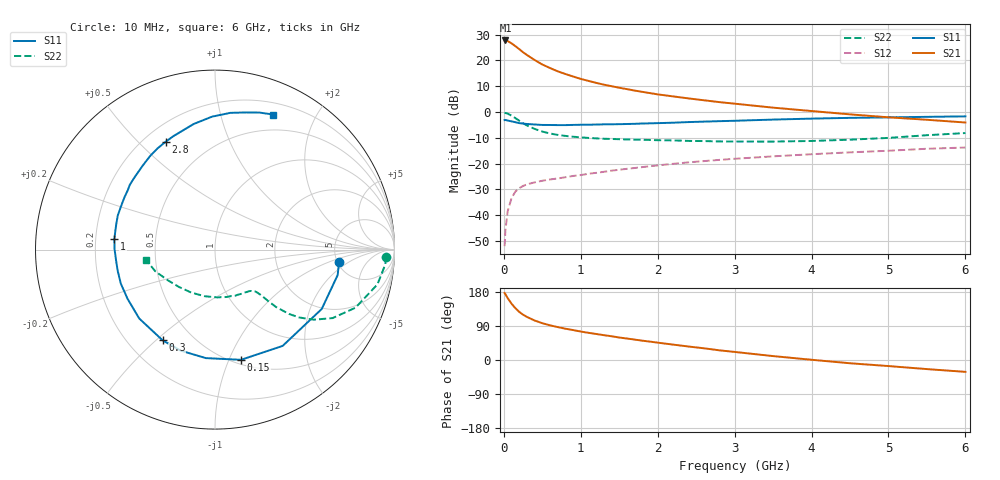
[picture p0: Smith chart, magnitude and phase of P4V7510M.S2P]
! SIEMENS Small Signal Semiconductors
! BFP182
! Si NPN RF Bipolar Junction Transistor in SOT143
! VCE = 0.75 V  IC = 10 mA
! Common Emitter S-Parameters:  March  1996
# GHz  S  MA  R  50
!  f  S11  S21  S12  S22
! GHz  MAG  ANG  MAG  ANG  MAG  ANG  MAG  ANG
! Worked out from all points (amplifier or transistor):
!   36 points, 10 MHz to 6 GHz, reference 50 ohm
!   highest |S21| = 27.7 dB at 20 MHz (marker M1)
!   |S21| within 3 dB of that: start of sweep to 184.4 MHz
!   unconditionally stable (mu >= 1): 793.1 MHz to end of sweep
!   at 250 MHz: K = 0.41, MSG = 25.9 dB, |S12| = -28.7 dB
!   at 1.4 GHz: K = 1.27, MAG = 13.2 dB, |S12| = -22.8 dB
!   at 6 GHz: K = 1.12, MAG = 2.7 dB, |S12| = -13.8 dB
!   S11 on the Smith chart (normalised r, x): 10 MHz: 5.15, -1.39; 150 MHz: 0.54, -1.11; 300 MHz: 0.34, -0.53; 1 GHz: 0.28, +0.05; 2.8 GHz: 0.28, +0.61; 6 GHz: 0.32, +1.47
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0.01  0.6941 -5.8  24.21 176.8  0.0025 86.0  0.9538 -2.4
0.02  0.6981 -11.7  24.25 173.7  0.005 83.0  0.9523 -5.0
0.05  0.6805 -29.1  23.59 163.3  0.0119 77.6  0.9255 -12.1
0.1  0.6557 -54.9  21.3 148.6  0.0213 65.2  0.8467 -22.5
0.15  0.631 -76.7  18.8 136.7  0.0286 56.6  0.7585 -30.2
0.2  0.6067 -94.8  16.48 127.0  0.0332 50.5  0.6757 -35.3
0.25  0.5946 -108.9  14.31 119.5  0.0367 45.9  0.6021 -38.9
0.3  0.5836 -120.0  12.7 113.7  0.0395 43.6  0.5461 -41.0
0.4  0.5706 -137.7  10.13 104.2  0.0431 40.2  0.4687 -43.2
0.5  0.559 -150.6  8.297 97.1  0.0463 39.1  0.4161 -44.0
0.6  0.5579 -160.1  7.093 91.5  0.0491 39.0  0.3817 -44.4
0.7  0.5548 -167.8  6.114 86.9  0.0513 39.6  0.3588 -44.8
0.8  0.5546 -174.1  5.431 82.6  0.0542 39.5  0.3427 -45.2
1  0.5637 173.8  4.363 75.1  0.0597 40.5  0.3212 -46.4
1.1  0.5651 169.2  3.99 71.7  0.0633 41.0  0.3133 -47.5
1.5  0.5782 153.4  2.939 59.3  0.0757 41.7  0.296 -52.7
2.2  0.6177 130.6  1.999 40.6  0.0986 39.4  0.2804 -66.4
2.8  0.6612 114.5  1.549 25.6  0.1175 35.7  0.2678 -81.7
3.5  0.71 99.6  1.209 10.3  0.1376 30.3  0.2661 -102.9
4.5  0.7667 83.6  0.896 -8.6  0.1645 22.4  0.2895 -134.2
5.5  0.8027 72.0  0.704 -24.0  0.1931 14.6  0.3536 -160.0
6  0.8196 66.6  0.623 -31.3  0.2041 9.5  0.3893 -171.6
